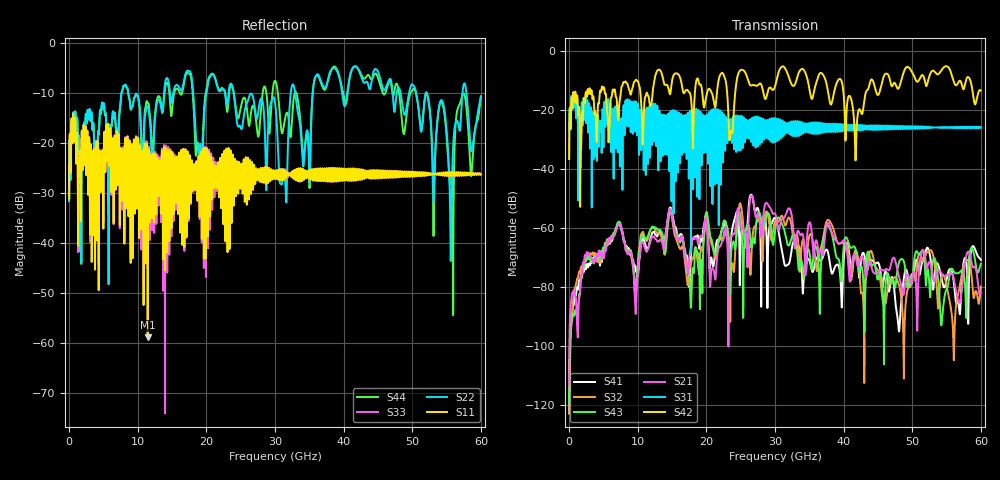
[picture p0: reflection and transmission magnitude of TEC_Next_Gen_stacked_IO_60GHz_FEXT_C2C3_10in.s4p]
!! CHANNEL DESCRIPTION:  Next Generation 28Gbps Press-fit Stacked I/O Connector
!!  with 10" 5-6-5 Megtron 6 Stripline trace on host side and 1.25" 7-5-7 Megtron 6 Microstrip trace on plug side
!! HOST PCB DESCRIPTION:  PCB thickness 3.425 mm
!!  26 Layer Board, 15 GND planes, 4 Layer route-out on Layers 7,11,17,21, 8mil stub on vias
!!  Pairs on following layers
!!  Layer 07 - A02A03 A14A15 D05D06
!!  Layer 11 - D020D3 C05C06 D14D15
!!  Layer 17 - C02C03 B05B06 C14C15
!!  Layer 21 - B02B03 A05A06 B14B15
!! CONNECTOR DESCRIPTION:  Next Generation 28Gbps Press-fit Stacked I/O Connector
!! PLUG-IN CARD DESCRIPTION:  PCB thickness 1mm thick
!!  6 Layer Board, 4 GND planes, 0.35 x 1.4mm mating pads
!!  Micro-strip diff traces referenced to GND plane 3mils down, 2nd GND plane 17mils from top of board
!!  PCB GND planes are symmetric
!! MODEL DESCRIPTION: TE Connectivity S-parameter model produced from Macro-model, Extracted .s4p FEXT (Victim B05B06 - Aggressor C02C03)
!! MODEL DATE: 5/15/2014 CR32f, FPR23
!! MODEL STATUS: Developmental
!! MODEL GEOMETRY: 4 Rows - Rows A, B, C, D. 3 pairs in each row, 12 total pairs
!! MODEL FREQUENCY RANGE: DC to 60 GHz in 10 MHz frequency steps
!! MODEL EDGE RATE LIMITATION: 8.33 ps (Using conservative 0.5/Fmax rule of thumb)
!! TIME-DOMAIN TRANSFORM CAUTIONS:
!! 1.) Do not simulate transient edge rates faster than the number listed above.  Edge
!!  rates faster than this number contain significant spectral content at frequencies
!!  above the model's highest frequency.
!! 2.) Even when simulating edge rates that are slower than the number listed above, be
!!  aware that the best time resolution possible with a direct iFFT is (1 / 2Fmax).
!!  As a result, time resolution is typically not adequate for most time-domain
!!  simulations unless tricks such as frequency-domain zero-padding and windowing are
!!  used to minimize leakage and aliasing.
!! 3.) Because the model has a uniform frequency step, a direct iFFT will result in an
!!  impulse that that has a time length given by either (1 / Fstep) or (1 / 2Fstep),
!!  depending on the transform being used.  Care has been taken in selecting the
!!  frequency step to ensure a settled impulse response for the model.  Therefore,
!!  convolution with the model's impulse response should present no issues.  However,
!!  if directly concatenating s-parameter models in the frequency domain a user must
!!  either interpolate necessary interim frequencies or complete impulse response
!!  zero-padding.  Impulse response zero-padding is more difficult, but more accurate.
!! PORT DEFINITIONS:
!! Port  1  ----->  Host C02		B05 Module <-----  Port  2
!! Port  3  ----->  Host C03		B06 Module <-----  Port  4
! Touchstone data
! Created: 29-Sep-2014 by IdEM R2011 (7.0.3)
# Hz S MA R 50
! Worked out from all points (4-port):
!   6000 points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, 10 MHz to 60 GHz, reference 50 ohm
!   strongest paths, dB at 10 MHz, 15.01 GHz, 30.01 GHz, 45.01 GHz, 60 GHz:
!     S42: -36.6, -10.1, -12.0, -14.9, -13.4
!     S31: -36.0, -22.9, -30.8, -25.5, -25.8
!     S21: -113.3, -55.9, -55.1, -75.2, -82.0
!     S43: -119.5, -56.0, -60.8, -77.4, -72.1
!     S32: -122.8, -56.8, -57.7, -74.4, -79.8
!     S41: -122.8, -54.7, -56.6, -71.7, -70.8
!   lowest |S11| = -58.8 dB at 11.46 GHz (marker M1), VSWR 1.00, Z = 50.1 + j0.0219 ohm
!   |S11| at or under -10 dB: start of sweep to end of sweep
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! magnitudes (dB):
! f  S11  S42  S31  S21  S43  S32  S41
! 10 MHz  -31.1  -36.6  -36.0  -113.3  -119.5  -122.8  -122.8
! 11.46 GHz  -58.8  -15.0  -29.3  -67.3  -62.7  -63.7  -66.8
! 26.61 GHz  -24.6  -11.6  -27.0  -48.9  -66.5  -67.1  -48.8
! 34.12 GHz  -26.1  -6.2  -27.6  -62.8  -75.6  -64.0  -80.4
! 41.75 GHz  -27.2  -36.8  -25.6  -69.7  -67.2  -67.8  -67.6
! 55.58 GHz  -26.3  -6.9  -26.0  -75.4  -74.4  -86.4  -74.0
! 60 GHz  -26.3  -13.4  -25.8  -82.0  -72.1  -79.8  -70.8
